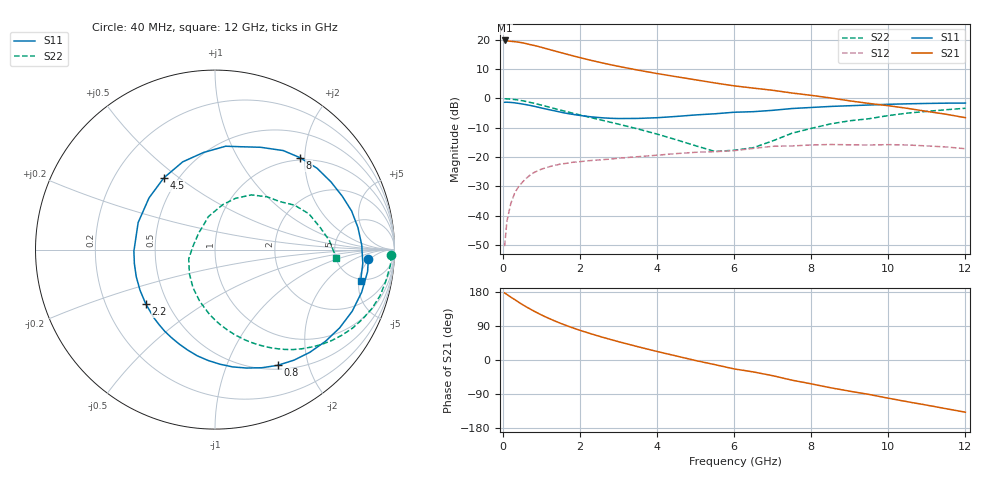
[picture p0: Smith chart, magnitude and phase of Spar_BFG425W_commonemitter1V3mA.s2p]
! Filename: 13bfg425.001
! BFG425W Field C1
! V1=8.203E-001V,V2=1.000E+000V, I1=4.157E-005A, I2=3.000E-003A
# GHz  S  MA  R 50
!  S11  S21  S12  S22
!Freq(GHz)  Mag  Ang  Mag  Ang  Mag  Ang  Mag  Ang
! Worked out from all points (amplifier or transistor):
!   44 points, 40 MHz to 12 GHz, reference 50 ohm
!   highest |S21| = 19.7 dB at 40 MHz (marker M1)
!   |S21| within 3 dB of that: start of sweep to 1.177 GHz
!   unconditionally stable (mu >= 1): 2.797 GHz to end of sweep
!   at 700 MHz: K = 0.24, MSG = 22.3 dB, |S12| = -26.2 dB
!   at 2.4 GHz: K = 0.86, MSG = 16.9 dB, |S12| = -21.1 dB
!   at 12 GHz: K = 1.63, MAG = 0.7 dB, |S12| = -17.2 dB
!   S11 on the Smith chart (normalised r, x): 40 MHz: 11, -4; 800 MHz: 0.55, -1.53; 2.2 GHz: 0.38, -0.30; 4.5 GHz: 0.42, +0.44; 8 GHz: 0.95, +1.90; 12 GHz: 4.69, -5.29
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0.04  0.856 -3.5  9.716 176.9  0.003 79.7  0.983 -1.9
0.1  0.859 -8.2  9.528 173.0  0.008 85.1  0.981 -5.1
0.2  0.851 -16.2  9.396 165.9  0.016 79.4  0.968 -10.5
0.3  0.838 -24.2  9.271 159.6  0.024 74.5  0.955 -15.6
0.5  0.8 -39.7  8.871 146.4  0.037 64.9  0.909 -25.1
0.6  0.779 -47.3  8.579 140.4  0.043 60.4  0.883 -29.6
0.8  0.733 -61.6  7.994 129.1  0.054 52.3  0.824 -38.0
0.9  0.708 -68.4  7.711 123.8  0.058 48.7  0.794 -41.8
1.1  0.661 -81.4  7.104 113.9  0.065 42.3  0.735 -48.7
1.5  0.58 -105.2  6.024 96.5  0.076 32.0  0.627 -60.6
1.8  0.534 -121.7  5.339 85.2  0.081 26.1  0.559 -68.2
2.2  0.49 -142.0  4.586 71.7  0.086 19.9  0.483 -77.4
2.6  0.464 -161.0  3.988 59.5  0.09 15.0  0.418 -86.2
3  0.452 -178.9  3.507 48.3  0.095 10.8  0.362 -94.9
3.5  0.454 160.6  3.03 35.0  0.101 5.9  0.3 -106.6
4.5  0.491 125.5  2.336 10.5  0.114 -4.0  0.196 -136.7
5.5  0.545 96.7  1.828 -12.3  0.123 -15.4  0.124 171.1
6.5  0.592 75.4  1.493 -31.5  0.14 -22.8  0.144 119.2
8  0.698 47.1  1.124 -63.0  0.16 -47.0  0.307 68.3
8.5  0.727 38.6  1.015 -73.2  0.163 -55.7  0.366 56.4
10.5  0.806 8.7  0.674 -110.2  0.16 -88.4  0.56 20.9
12  0.83 -12.2  0.467 -137.7  0.138 -117.5  0.677 -3.8
